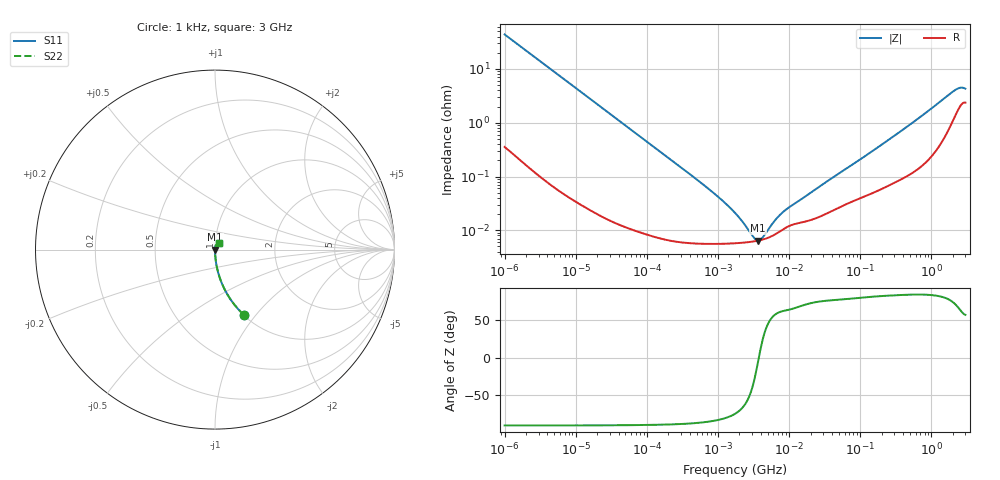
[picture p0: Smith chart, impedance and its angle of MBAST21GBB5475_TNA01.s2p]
! MBAST21GBB5475_TNA01  S-PARAMETER MODEL  ( Standard Model )
! Model Generated by TAIYO YUDEN Corporation (http://www.ty-top.com)
! Version 1.0
! TAIYO YUDEN Control No. 220601
! Copyright(c) 2013 TAIYO YUDEN CO.,LTD. All Rights Reserved.
! Product Description (link to TY-COMPAS)
! https://ds.yuden.co.jp/TYCOMPAS/or/detail?pn=MBAST21GBB5475KTNA01&u=M
! Products Name : Multilayer Ceramic Capacitors
! Characteristics :
!  Capacitance : 4.7 [uF] , Rated Voltage : 25 [V] , TCC : X5R
!  Case Size : 2.0 x 1.25 / 0.079 x 0.049 [mm/inch] , Thickness : 1.25 / 0.049 [mm/inch]
!  (Conditions: Temperature = 25 [degC] , DC Bias Voltage = 0 [V])
! External Node Assignments :
!  1  o---| |---o  2
! GND o---------o GND
! Frequency Range : 1kHz  -  3GHz  [ 401 STEP ]
# MHZ S RI R 50
! Freq[MHz].  S11 Real  S11 Imag  S21 Real  S21 Imag  S12 Real  S12 Imag  S22 Real  S22 Imag
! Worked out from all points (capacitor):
!   401 points, 1 kHz to 3 GHz, reference 50 ohm
!   read as one part in series: C = 3.62 uF near 1.077 kHz
!   lowest |Z| = 6.44 mohm at 3.651 MHz (marker M1)
!   series resonance near 3.746 MHz, so ESL is about 500 pH
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0.001  0.1634 -0.3657  0.8366 0.3657  0.8366 0.3657  0.1634 -0.3657
0.001685  0.0654 -0.2435  0.9346 0.2435  0.9346 0.2435  0.0654 -0.2435
0.003177  0.0198 -0.136  0.9802 0.136  0.9802 0.136  0.0198 -0.136
0.005768  0.00637 -0.0761  0.9936 0.0761  0.9936 0.0761  0.00637 -0.0761
0.01216  0.00162 -0.0364  0.9984 0.0364  0.9984 0.0364  0.00162 -0.0364
0.147855  8.06e-05 -0.00303  0.9999 0.00303  0.9999 0.00303  8.06e-05 -0.00303
0.791611  5.6e-05 -0.000542  0.9999 0.000542  0.9999 0.000542  5.6e-05 -0.000542
1.238299  5.62e-05 -0.000323  0.9999 0.000323  0.9999 0.000323  5.62e-05 -0.000323
1.732051  5.73e-05 -0.000203  0.9999 0.000203  0.9999 0.000203  5.73e-05 -0.000203
2.709407  6.03e-05 -7.86e-05  0.9999 7.86e-05  0.9999 7.86e-05  6.03e-05 -7.86e-05
2.919173  6.11e-05 -6e-05  0.9999 6e-05  0.9999 6e-05  6.11e-05 -6e-05
3.651041  6.41e-05 -6.06e-06  0.9999 6.06e-06  0.9999 6.06e-06  6.41e-05 -6.06e-06
4.919932  7.15e-05 6.56e-05  0.9999 -6.56e-05  0.9999 -6.56e-05  7.15e-05 6.56e-05
5.30084  7.44e-05 8.39e-05  0.9999 -8.39e-05  0.9999 -8.39e-05  7.44e-05 8.39e-05
6.881678  8.96e-05 0.000149  0.9999 -0.000149  0.9999 -0.000149  8.96e-05 0.000149
8.606987  0.000108 0.000204  0.9999 -0.000204  0.9999 -0.000204  0.000108 0.000204
21.06097  0.000158 0.000498  0.9998 -0.000498  0.9998 -0.000498  0.000158 0.000498
256.0921  0.000709 0.00487  0.9993 -0.00487  0.9993 -0.00487  0.000709 0.00487
675.1638  0.00158 0.0123  0.9984 -0.0123  0.9984 -0.0123  0.00158 0.0123
2066.299  0.0131 0.0364  0.9869 -0.0364  0.9869 -0.0364  0.0131 0.0364
2489.759  0.0207 0.0384  0.9793 -0.0384  0.9793 -0.0384  0.0207 0.0384
3000  0.0244 0.0342  0.9756 -0.0342  0.9756 -0.0342  0.0244 0.0342
